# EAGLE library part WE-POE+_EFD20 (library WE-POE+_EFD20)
Transformer for Power-over-Ethernet WE-PoE+ - Designed to meet 30W PoE+ objectives of IEEE802.3at - Frequency range: 250-400 kHz - Insulation voltage 1,5 kVAC/1 min - Input voltages 36V till 72V -- PoE+ Powered devices -- Ip phones -- WLAN-Access point -- Security cameras
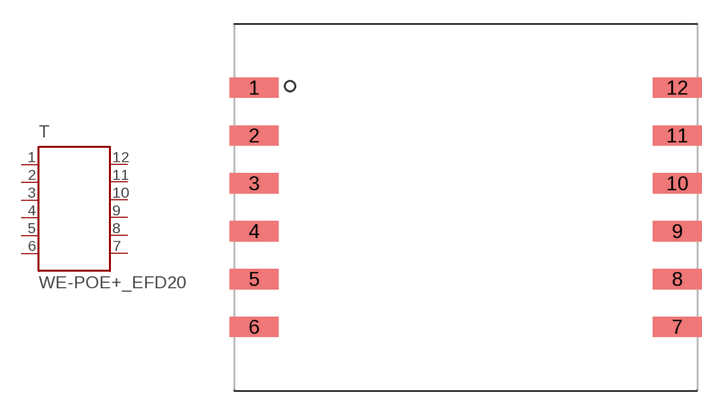
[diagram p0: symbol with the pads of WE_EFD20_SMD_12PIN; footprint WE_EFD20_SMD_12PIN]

Designator prefix T

## WE-POE+_EFD20, WE-POE+_EFD20-749119433 (MPN: 749119433; OC_FARNELL: 1849019; OC_NEWARK: 13T9813; PACKAGE: EFD20; SUPPLIER: Wuerth Elektronik), WE-POE+_EFD20-749119450 (MPN: 749119450; OC_FARNELL: 1849020; OC_NEWARK: 13T9814; PACKAGE: EFD20; SUPPLIER: Wuerth Elektronik), WE-POE+_EFD20-7491194501 (MPN: 7491194501; OC_FARNELL: 1849021; OC_NEWARK: 13T9815; PACKAGE: EFD20; SUPPLIER: Wuerth Elektronik), WE-POE+_EFD20-7491194912 (MPN: 7491194912; OC_FARNELL: 1849023; OC_NEWARK: 13T9816; PACKAGE: EFD20; SUPPLIER: Wuerth Elektronik), WE-POE+_EFD20-750310925 (MPN: 750310925; OC_FARNELL: 1849018; OC_NEWARK: 13T9831; PACKAGE: EFD20; SUPPLIER: Wuerth Elektronik), WE-POE+_EFD20-750310926 (MPN: 750310926; OC_FARNELL: 1849022; OC_NEWARK: 13T9832; PACKAGE: EFD20; SUPPLIER: Wuerth Elektronik), WE-POE+_EFD20-750310927 (MPN: 750310927; OC_FARNELL: 1849024; OC_NEWARK: 13T9833; PACKAGE: EFD20; SUPPLIER: Wuerth Elektronik)  [WE_EFD20_SMD_12PIN]
1  1  pas
2  2  pas
3  3  pas
4  4  pas
5  5  pas
6  6  pas
7  7  pas
8  8  pas
9  9  pas
10  10  pas
11  11  pas
12  12  pas

## Footprint WE_EFD20_SMD_12PIN (pad centres in mm)
Transformer, EFD20 SMD 12 Pin
smd 3.05 x 1.27: 1 -13.26,7.5; 2 -13.26,4.5; 3 -13.26,1.5; 4 -13.26,-1.5; 5 -13.26,-4.5; 6 -13.26,-7.5; 7 13.26,-7.5; 8 13.26,-4.5; 9 13.26,-1.5; 10 13.26,1.5; 11 13.26,4.5; 12 13.26,7.5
